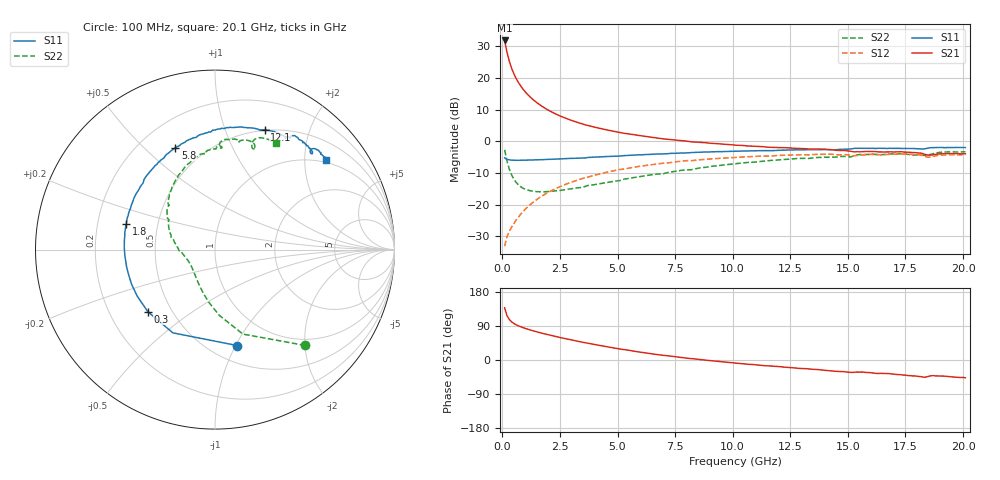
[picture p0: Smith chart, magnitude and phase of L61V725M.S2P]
!  Infineon Technologies AG
! BFR380L3 , PF131585-7, No.6, Th 09.10.01, soldered on pcb-board, measured with PP GSG850
!  Vce=1.75 V,  Ic=25.0 mA
! Common Emitter S-Parameters:  15. November 2001
#  GHz  S  MA  R  50
! f  S11  S21  S12  S22
! GHz  Mag  Ang  Mag  Ang  Mag  Ang  Mag  Ang
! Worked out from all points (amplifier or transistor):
!   201 points, 100 MHz to 20.1 GHz, reference 50 ohm
!   highest |S21| = 31.8 dB at 100 MHz (marker M1)
!   |S21| within 3 dB of that: start of sweep to 183.2 MHz
!   unconditionally stable (mu >= 1): 1.25 GHz to 4.447 GHz
!   at 3.4 GHz: K = 1.02, MAG = 8.0 dB, |S12| = -11.9 dB
!   at 10.1 GHz: K = 0.96, MSG = 1.9 dB, |S12| = -5.1 dB
!   at 20.1 GHz: K = 0.99, MSG = 0.1 dB, |S12| = -4.2 dB
!   S11 on the Smith chart (normalised r, x): 100 MHz: 0.66, -1.01; 300 MHz: 0.37, -0.34; 1.8 GHz: 0.33, +0.13; 5.8 GHz: 0.35, +0.63; 12.1 GHz: 0.49, +1.38; 20.1 GHz: 0.92, +2.54
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0.1  0.5487 -77.0  39.07 137.9  0.02214 60.9  0.7338 -46.7
0.2  0.5199 -116.9  25.79 117.5  0.03097 55.1  0.4958 -71.7
0.3  0.5096 -137.3  18.59 107.3  0.0379 55.3  0.3681 -86.1
0.4  0.5052 -149.3  14.38 100.9  0.04396 57.0  0.2967 -96.5
0.5  0.5032 -157.5  11.69 96.5  0.05028 59.5  0.2533 -104.7
0.6  0.5013 -163.6  9.826 93.0  0.05715 60.9  0.225 -111.4
0.7  0.5018 -168.6  8.481 90.1  0.06388 62.3  0.2056 -117.4
0.8  0.5015 -172.4  7.461 87.5  0.07084 63.5  0.1918 -122.4
1  0.5042 -178.9  6.016 83.2  0.08493 64.7  0.1751 -131.0
1.2  0.5065 176.0  5.043 79.4  0.09918 65.2  0.1663 -137.9
1.5  0.5115 169.2  4.071 74.2  0.1209 65.1  0.1604 -145.9
1.8  0.5147 163.7  3.421 69.5  0.1427 64.2  0.1597 -152.5
2.5  0.5281 151.9  2.522 59.5  0.192 60.9  0.1678 -164.0
3.5  0.5455 137.6  1.868 46.6  0.2606 54.5  0.188 -176.1
4.6  0.5751 124.2  1.498 34.4  0.3296 47.0  0.226 170.9
5.8  0.6094 111.3  1.257 22.5  0.3951 38.6  0.2715 158.3
6.8  0.6313 101.9  1.118 13.8  0.4444 31.3  0.3054 147.7
10.1  0.6997 77.8  0.8704 -8.0  0.5569 9.8  0.4425 120.1
12.1  0.7229 67.5  0.7963 -17.9  0.6003 -1.9  0.5117 104.7
13.5  0.7382 60.6  0.7587 -24.6  0.6176 -10.2  0.547 95.2
16.8  0.7752 48.2  0.6818 -36.0  0.6227 -25.7  0.6299 75.6
20.1  0.7979 38.9  0.6366 -47.0  0.6166 -39.1  0.6844 60.2
